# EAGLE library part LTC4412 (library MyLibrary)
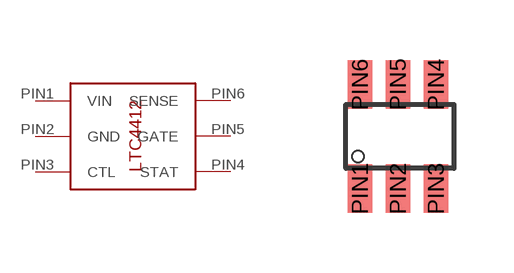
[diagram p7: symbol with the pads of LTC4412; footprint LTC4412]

Designator prefix -

## LTC4412  [LTC4412]
PIN1  VIN
PIN2  GND
PIN3  CTL
PIN4  STAT
PIN5  GATE
PIN6  SENSE

## Footprint LTC4412 (pad centres in mm)
smd 0.62 x 1.22: PIN1 -0.95,-1.3; PIN2 0,-1.3; PIN3 0.95,-1.3; PIN4 0.95,1.3; PIN5 0,1.3; PIN6 -0.95,1.3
